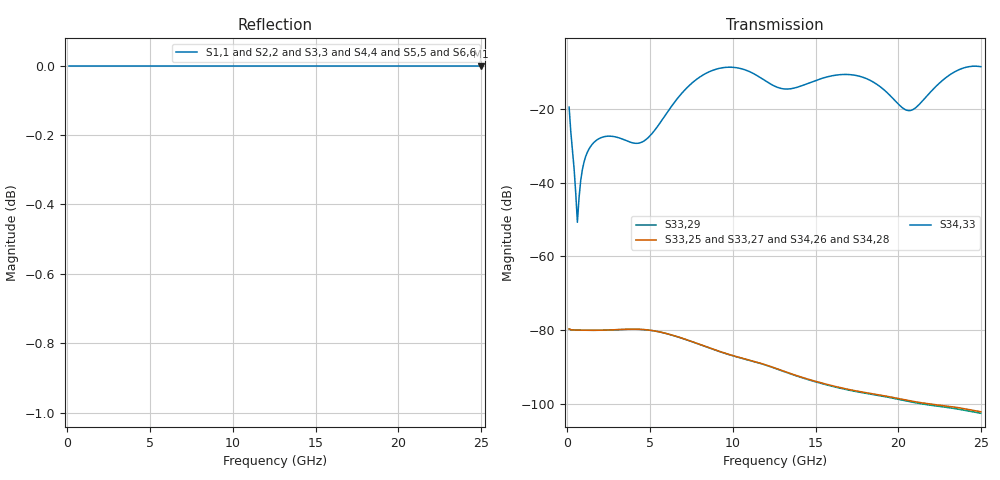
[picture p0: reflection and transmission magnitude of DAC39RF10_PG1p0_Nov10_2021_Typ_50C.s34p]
! Touchstone Ver. 1.0
! Number of ports is 34
# Hz	S	RI	R	50.000000
! SCATTERING PARAMETERS  :
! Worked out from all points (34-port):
!   250 points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, 100 MHz to 25 GHz, reference 50 ohm
!   strongest paths, dB at 100 MHz, 6.3 GHz, 12.6 GHz, 18.8 GHz, 25 GHz:
!     S34,33: -19.5, -19.2, -13.9, -13.6, -8.5
!     S33,25: -79.7, -81.3, -90.4, -97.6, -102.2
!     S33,27: -79.7, -81.4, -90.4, -97.7, -102.4
!     S34,26: -79.7, -81.3, -90.5, -97.7, -102.5
!     S33,29: -79.7, -81.4, -90.5, -97.8, -102.6
!     S34,28: -79.7, -81.3, -90.5, -97.8, -102.7
!   lowest |S11| = 0.0 dB at 25 GHz (marker M1)
!   |S11| at or under -10 dB: nowhere
